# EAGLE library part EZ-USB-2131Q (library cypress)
Microcontroller with USB port
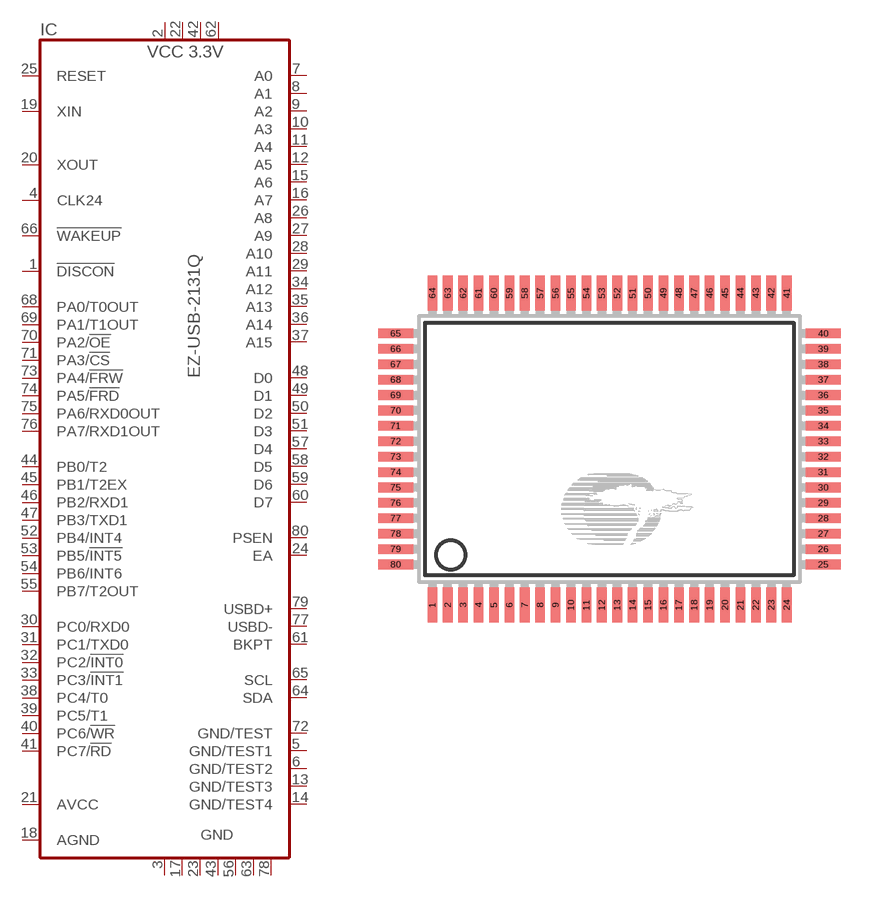
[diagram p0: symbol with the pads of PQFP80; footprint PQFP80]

Designator prefix IC

## EZ-USB-2131Q (OC_FARNELL: unknown; OC_NEWARK: unknown)  [PQFP80]
1  !DISCON  out
2  VCC3.3  pwr
3  GND  pwr
4  CLK24  out
5  GND/TEST1  pwr
6  GND/TEST2  pwr
7  A0  out
8  A1  out
9  A2  out
10  A3  out
11  A4  out
12  A5  out
13  GND/TEST3  pwr
14  GND/TEST4  pwr
15  A6  out
16  A7  out
17  GND  pwr
18  AGND  pwr
19  XIN  in
20  XOUT  out
21  AVCC  pwr
22  VCC3.3  pwr
23  GND  pwr
24  EA  in
25  RESET  in
26  A8  out
27  A9  out
28  A10  out
29  A11  out
30  PC0/RXD0
31  PC1/TXD0
32  PC2/!INT0
33  PC3/!INT1
34  A12  out
35  A13  out
36  A14  out
37  A15  out
38  PC4/T0
39  PC5/T1
40  PC6/!WR
41  PC7/!RD
42  VCC3.3  pwr
43  GND  pwr
44  PB0/T2
45  PB1/T2EX
46  PB2/RXD1
47  PB3/TXD1
48  D0  hiz
49  D1  hiz
50  D2  hiz
51  D3  hiz
52  PB4/INT4
53  PB5/!INT5
54  PB6/INT6
55  PB7/T2OUT
56  GND  pwr
57  D4  hiz
58  D5  hiz
59  D6  hiz
60  D7  hiz
61  BKPT  out
62  VCC3.3  pwr
63  GND  pwr
64  SDA  oc
65  SCL  oc
66  !WAKEUP  in
68  PA0/T0OUT
69  PA1/T1OUT
70  PA2/!OE
71  PA3/!CS
72  GND/TEST  pwr
73  PA4/!FRW
74  PA5/!FRD
75  PA6/RXD0OUT
76  PA7/RXD1OUT
77  USBD-  hiz
78  GND  pwr
79  USBD+  hiz
80  PSEN  out

## Footprint PQFP80 (pad centres in mm)
Plastic Quad Flat Package from micro-philips.lbr
smd 0.5 x 1.8: 1 -9.2,-8.1; 2 -8.4,-8.1; 3 -7.6,-8.1; 4 -6.8,-8.1; 5 -6,-8.1; 6 -5.2,-8.1; 7 -4.4,-8.1; 8 -3.6,-8.1; 9 -2.8,-8.1; 10 -2,-8.1; 11 -1.2,-8.1; 12 -0.4,-8.1; 13 0.4,-8.1; 14 1.2,-8.1; 15 2,-8.1; 16 2.8,-8.1; 17 3.6,-8.1; 18 4.4,-8.1; 19 5.2,-8.1; 20 6,-8.1; 21 6.8,-8.1; 22 7.6,-8.1; 23 8.4,-8.1; 24 9.2,-8.1; 41 9.2,8.1; 42 8.4,8.1; 43 7.6,8.1; 44 6.8,8.1; 45 6,8.1; 46 5.2,8.1; 47 4.4,8.1; 48 3.6,8.1; 49 2.8,8.1; 50 2,8.1; 51 1.2,8.1; 52 0.4,8.1; 53 -0.4,8.1; 54 -1.2,8.1; 55 -2,8.1; 56 -2.8,8.1; 57 -3.6,8.1; 58 -4.4,8.1; 59 -5.2,8.1; 60 -6,8.1; 61 -6.8,8.1; 62 -7.6,8.1; 63 -8.4,8.1; 64 -9.2,8.1
smd 1.8 x 0.5: 25 11.1,-6; 26 11.1,-5.2; 27 11.1,-4.4; 28 11.1,-3.6; 29 11.1,-2.8; 30 11.1,-2; 31 11.1,-1.2; 32 11.1,-0.4; 33 11.1,0.4; 34 11.1,1.2; 35 11.1,2; 36 11.1,2.8; 37 11.1,3.6; 38 11.1,4.4; 39 11.1,5.2; 40 11.1,6; 65 -11.1,6; 66 -11.1,5.2; 67 -11.1,4.4; 68 -11.1,3.6; 69 -11.1,2.8; 70 -11.1,2; 71 -11.1,1.2; 72 -11.1,0.4; 73 -11.1,-0.4; 74 -11.1,-1.2; 75 -11.1,-2; 76 -11.1,-2.8; 77 -11.1,-3.6; 78 -11.1,-4.4; 79 -11.1,-5.2; 80 -11.1,-6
